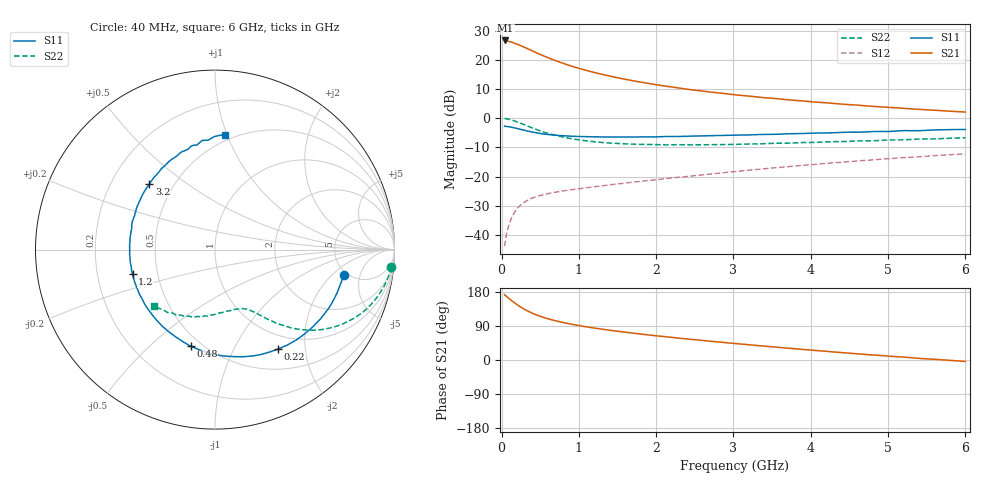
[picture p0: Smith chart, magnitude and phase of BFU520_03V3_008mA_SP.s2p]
! Filename:  P:\Prog\Test\Noise\ATS_data\Testdata_Net\03 Spar\BFU520_APG2013_37_A05_03p3V_008mA_SP_CM01_D.s2p
! Date/Time: Fri 26/Apr/2013 13:00:03
! BFU520_APG2013_37_A05_03p3V_1to20mA_SP_CM01_Bias5_R.s2p
! MDIF S-parameter v. bias file
! BFU520_APG2013_37_A05_03p3V_1to20mA_SP_CM01
! Date/time Tue Apr 23 14:11:50 2013
! VAR V_out= 3.3010
! VAR I_out= 7.9950
! VAR V_in= 0.8407
! VAR I_in= 0.0931
! Device data file deembeded for feedlines and parallel
! Original file: \03 Spar\BFU520_APG2013_37_A05_03p3V_008mA_SP_CM01_R.s2p
! Feed-files: PR047V01_250413_Feed1.s2p, PR047V01_250413_Feed2.s2p
! Parallel-file: PR047V01_250413_Par.s2p
# MHz S MA R 50
!  Freq-MHz  S11-mag  S11-arg  S21-mag  S21-arg  S12-mag  S12-arg  S22-mag  S22-arg
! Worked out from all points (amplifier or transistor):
!   98 points, 40 MHz to 6 GHz, reference 50 ohm
!   highest |S21| = 26.7 dB at 50 MHz (marker M1)
!   |S21| within 3 dB of that: start of sweep to 350.7 MHz
!   unconditionally stable (mu >= 1): 1.875 GHz to 4.122 GHz
!   at 300 MHz: K = 0.27, MSG = 26.5 dB, |S12| = -28.7 dB
!   at 1.6 GHz: K = 0.94, MSG = 17.8 dB, |S12| = -22.3 dB
!   at 6 GHz: K = 0.86, MSG = 7.2 dB, |S12| = -12.2 dB
!   S11 on the Smith chart (normalised r, x): 40 MHz: 4.62, -2.83; 220 MHz: 0.78, -1.52; 480 MHz: 0.44, -0.68; 1.2 GHz: 0.36, -0.13; 3.2 GHz: 0.37, +0.37; 6 GHz: 0.46, +0.99
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40  0.7301 -11.3  21.53 172.5  0.006392 84.8  0.9855 -5.7
50  0.727 -14.1  21.54 170.1  0.007955 83.4  0.9842 -7.1
120  0.7035 -33.1  20.39 158.4  0.01817 74.2  0.9389 -16.8
140  0.6944 -38.3  19.97 155.2  0.02079 71.9  0.9223 -19.3
180  0.677 -48.1  19.06 149.1  0.02565 67.5  0.8854 -23.9
220  0.6564 -57.6  18.24 143.4  0.02983 63.9  0.8453 -28.1
260  0.6378 -66.4  17.28 138.2  0.0335 60.6  0.8058 -31.8
320  0.6094 -78.5  15.95 131.3  0.03806 56.4  0.7481 -36.5
400  0.5788 -92.4  14.23 123.4  0.04277 52.5  0.6783 -41.2
480  0.5547 -104.2  12.74 117.0  0.04657 49.6  0.62 -45.0
600  0.5256 -119.2  10.93 108.9  0.05089 47.0  0.551 -49.1
700  0.5112 -129.2  9.696 103.5  0.05387 45.7  0.5076 -51.5
850  0.4962 -141.7  8.261 96.7  0.05797 45.0  0.4592 -54.4
1050  0.4836 -155.2  6.871 89.1  0.06293 45.0  0.4167 -57.6
1200  0.4793 -163.3  6.086 84.3  0.0667 45.5  0.3951 -59.6
1600  0.4752 179.1  4.649 73.3  0.07714 47.0  0.3634 -64.9
2050  0.4814 164.6  3.659 62.9  0.08946 48.5  0.351 -71.5
3100  0.5143 136.7  2.461 42.1  0.1244 49.4  0.3582 -88.4
3200  0.5169 134.9  2.395 40.2  0.1287 49.2  0.3608 -89.8
4100  0.5574 115.9  1.873 24.6  0.1635 46.2  0.3863 -105.2
5200  0.6128 96.7  1.476 7.7  0.2106 39.9  0.4257 -123.9
6000  0.6407 84.8  1.276 -3.9  0.2452 33.8  0.462 -137.3
